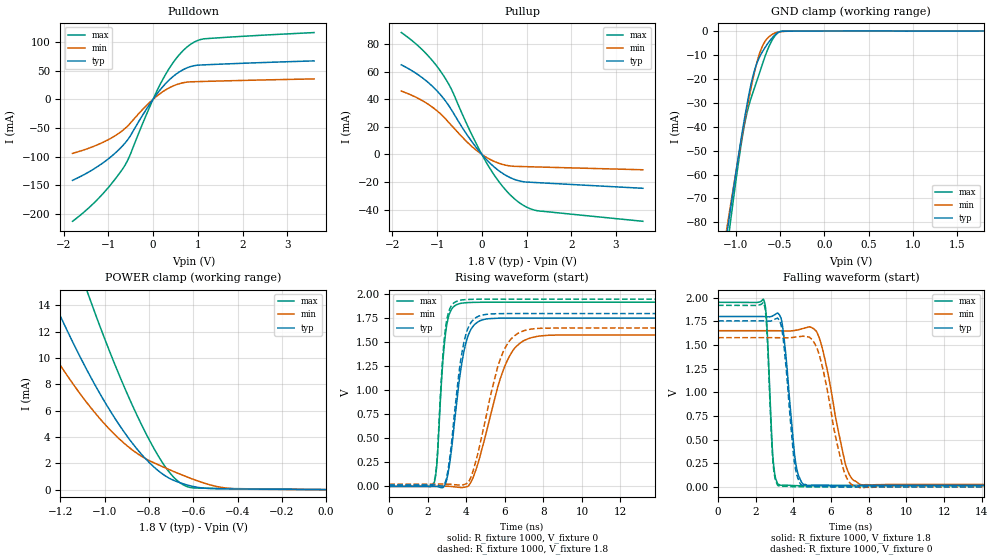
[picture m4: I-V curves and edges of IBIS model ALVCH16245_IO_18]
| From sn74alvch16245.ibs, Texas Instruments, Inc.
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[Model]   ALVCH16245_IO_18
Model_type  I/O
Vinl=0.5775
Vinh=1.2675
Enable   Active-Low
Vref =   0
Rref =   1000
Cref =   30p
Vmeas =   0.9
| variable   typ   min   max
C_comp   8.49pF   7.56pF   9.33pF
| C_pullup   9.56pF   8.05pF   10.45pF
| C_pulldown   12.46pF   9.75pF   16.07pF
| C_tri-state   8.49pF   7.56pF   9.33pF
[Temperature Range]   40   100   -40
| Ambient temperature   25   85   -40
[Voltage range]   1.8   1.65   1.95
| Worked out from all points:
|   slope of the pulldown table from 0 to 0.27 V, typ, clamps not added: 10.2 ohm
|   slope of the pullup table from 0 to 0.27 V, typ, clamps not added: 30.2 ohm
|   GND clamp passes 1 mA (typ) near -0.54 V on its own axis
|   POWER clamp passes 1 mA (typ) near -0.72 V on its own axis
|   rising waveform, R_fixture 1000, V_fixture 0: 20-80 % time 663ps typ, 1.31ns min, 365ps max; typ from 0 V to 1.75 V
|   falling waveform, R_fixture 1000, V_fixture 1.8: 20-80 % time 472ps typ, 942ps min, 256ps max; typ from 1.8 V to 0.016 V
|   rising waveform, R_fixture 1000, V_fixture 1.8: 20-80 % time 633ps typ, 1.16ns min, 354ps max; typ from 0.016 V to 1.8 V
|   falling waveform, R_fixture 1000, V_fixture 0: 20-80 % time 457ps typ, 939ps min, 251ps max; typ from 1.75 V to 0 V
[GND Clamp]
| ALVCH16245_IO_18
|   Voltage   I(typ)   I(min)   I(max)
-1.8V     -279.5mA   -258.7mA   -313.2mA
-1.09V    -82.31mA   -80.08mA   -88.64mA
-1.075V   -78.45mA   -76.58mA   -84.27mA
-1.055V   -73.35mA   -71.94mA   -78.51mA
-920mV    -40.76mA   -42.01mA   -43.09mA
-870mV    -30.11mA   -31.83mA   -33.72mA
-815mV    -20.23mA   -21.6mA    -26.7mA
-765mV    -13.84mA   -13.69mA   -21.2mA
-710mV    -9.381mA   -7.29mA    -15.07mA
-585mV    -2.692mA   -1.324mA   -3.554mA
-485mV    -106.2uA   -262.8uA   -133.2uA
1.8V      63.54pA    9.524uA    -22.72uA
[POWER Clamp]
| ALVCH16245_IO_18
|   Voltage   I(typ)   I(min)   I(max)
-1.8V     39.84mA    29.03mA    57.62mA
-1.39V    20.65mA    14.81mA    31.6mA
-1.245V   14.85mA    10.62mA    23.46mA
-1.08V    9.08mA     6.594mA    15.11mA
-1.065V   8.608mA    6.273mA    14.4mA
-940mV    5.06mA     3.946mA    8.929mA
-825mV    2.518mA    2.444mA    4.637mA
-735mV    1.142mA    1.715mA    1.939mA
-665mV    553.8uA    1.212mA    582uA
-610mV    273.2uA    844.7uA    148.5uA
-455mV    56.6uA     123.1uA    83uA
-16.28fV  63.54pA    290.7pA    36.64pA
[Pulldown]
| ALVCH16245_IO_18
|   Voltage   I(typ)   I(min)   I(max)
-1.8V     -141.4mA   -94.33mA   -212.9mA
-1.195V   -115mA     -77.76mA   -171mA
-905mV    -97.86mA   -66.26mA   -145mA
-665mV    -79.81mA   -53.39mA   -119.8mA
-530mV    -66.51mA   -43.55mA   -100.1mA
-105mV    -12.13mA   -7.634mA   -18.73mA
200mV     20.41mA    12.38mA    32.16mA
495mV     42.75mA    24.8mA     68.98mA
790mV     55.87mA    30.28mA    93.18mA
970mV     59.35mA    30.84mA    101.8mA
1.155V    60.2mA     31.26mA    105.7mA
3.6V      67.09mA    35.62mA    116.5mA
[Pullup]
| ALVCH16245_IO_18
|   Voltage   I(typ)   I(min)   I(max)
-1.8V     64.98mA    45.95mA    88.4mA
-1.305V   54.98mA    38.53mA    75.09mA
-1.09V    48.97mA    33.9mA     67.43mA
-900mV    42.35mA    28.69mA    59.27mA
-675mV    32.13mA    20.88mA    46.91mA
-280mV    11.84mA    7.43mA     18.08mA
120mV     -4.3mA     -2.474mA   -6.918mA
455mV     -13.55mA   -7.178mA   -22.84mA
795mV     -18.85mA   -8.713mA   -33.97mA
1.025V    -20.11mA   -8.923mA   -38.62mA
1.255V    -20.5mA    -9.129mA   -40.95mA
3.6V      -24.58mA   -11.14mA   -48.53mA
[Ramp]
| ALVCH16245_IO_18
| variable   typ   min   max
dV/dt_r   1.06/6.83E-10   0.95/1.36E-09   1.15/3.68E-10
dV/dt_f   1.09/4.88E-10   1.00/9.78E-10   1.18/2.69E-10
R_load = 1000
[Rising Waveform]
| ALVCH16245_IO_18
R_fixture =   1000
C_fixture =   0
L_fixture =   0
V_fixture =   0
V_fixture_min = 0
V_fixture_max = 0
|   Time   V(typ)   V(min)   V(max)
0s        343.1pV    1.757nV    237.2pV
2.32ns    600.7uV    262.6uV    27.99mV
2.485ns   -1.208mV   1.091mV    267mV
2.75ns    -14.96mV   1.665mV    1.212V
2.96ns    52.11mV    1.587mV    1.649V
3.72ns    1.224V     -11.64mV   1.907V
4.595ns   1.712V     232.6mV    1.917V
6.12ns    1.753V     1.308V     1.918V
7.7ns     1.753V     1.563V     1.918V
50ns      1.753V     1.576V     1.918V
[Falling Waveform]
| ALVCH16245_IO_18
R_fixture =   1000
C_fixture =   0
L_fixture =   0
V_fixture =   1.8
V_fixture_min = 1.65
V_fixture_max = 1.95
|   Time   V(typ)   V(min)   V(max)
0s        1.8V       1.65V      1.95V
2.445ns   1.8V       1.65V      1.966V
2.935ns   1.81V      1.65V      264.7mV
3.33ns    1.791V     1.649V     16.45mV
4.125ns   254.1mV    1.655V     12.71mV
4.755ns   15.68mV    1.686V     11.26mV
5.495ns   18.96mV    1.496V     11.06mV
6.82ns    16.02mV    204.9mV    11.03mV
7.64ns    15.91mV    20.87mV    11.05mV
50ns      15.9mV     23.5mV     11.07mV
[Rising Waveform]
| ALVCH16245_IO_18
R_fixture =   1000
C_fixture =   0
L_fixture =   0
V_fixture =   1.8
V_fixture_min = 1.65
V_fixture_max = 1.95
|   Time   V(typ)   V(min)   V(max)
0s        15.9mV     23.5mV     11.07mV
2.32ns    16.08mV    23.75mV    41.22mV
2.48ns    14.28mV    24.36mV    281.8mV
2.745ns   2.298mV    24.46mV    1.257V
2.945ns   64.86mV    23.97mV    1.683V
3.685ns   1.281V     14.09mV    1.938V
4.335ns   1.73V      151mV      1.949V
5.91ns    1.8V       1.399V     1.95V
7.3ns     1.8V       1.636V     1.95V
50ns      1.8V       1.65V      1.95V
[Falling Waveform]
| ALVCH16245_IO_18
R_fixture =   1000
C_fixture =   0
L_fixture =   0
V_fixture =   0
V_fixture_min = 0
V_fixture_max = 0
|   Time   V(typ)   V(min)   V(max)
0s        1.753V     1.576V     1.918V
2.44ns    1.753V     1.576V     1.932V
2.925ns   1.762V     1.576V     242.6mV
3.315ns   1.73V      1.576V     4.687mV
4.07ns    240.1mV    1.581V     1.576mV
4.62ns    2.674mV    1.59V      187.8uV
5.4ns     2.642mV    1.377V     -13.71uV
6.7ns     23.17uV    158.2mV    -38.57uV
7.565ns   -9.425uV   -9.494mV   -18.67uV
50ns      363.2nV    710.5nV    164.2nV
